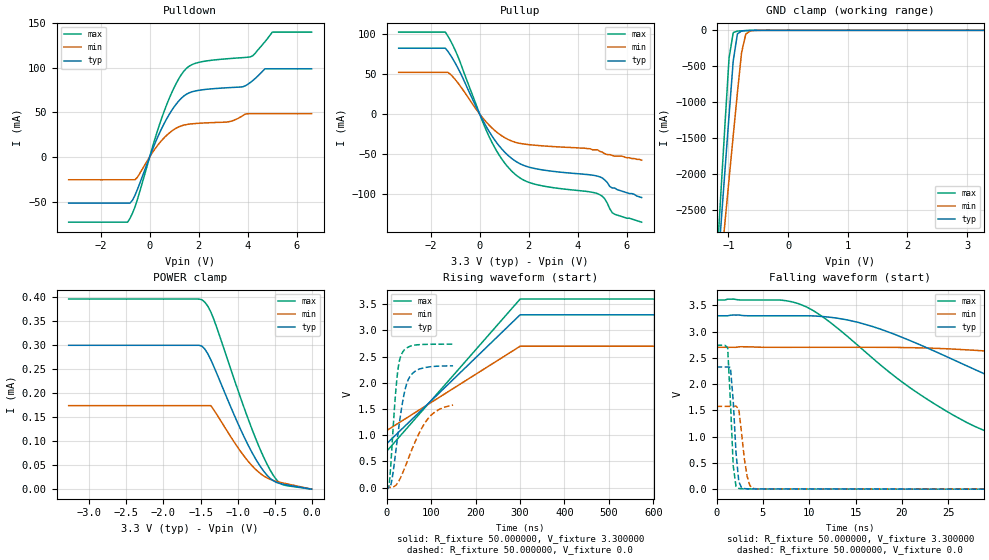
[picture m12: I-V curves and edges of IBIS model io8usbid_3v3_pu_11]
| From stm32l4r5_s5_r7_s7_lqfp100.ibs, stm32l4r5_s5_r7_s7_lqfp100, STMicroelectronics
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|   Model io8usbid_3v3_pu_11
[Model]  io8usbid_3v3_pu_11
Model_type I/O
Polarity   Non-Inverting
Enable   Active-Low
Vinl =   0.990000V
Vinh =   2.310000V
Vmeas =  1.650000V
Cref =   100.000000nF
Rref =   1.000000k
Vref =   3.300000V
C_comp   2.116400pF   2.092700pF   2.152900pF
[Temperature Range]   25.000000   0.125000k   -40.000000
[Pullup Reference]   3.300000V   2.700000V   3.600000V
[Pulldown Reference]   0.0V   0.0V   0.0V
[POWER Clamp Reference]   3.300000V   2.700000V   3.600000V
[GND Clamp Reference]   0.0V   0.0V   0.0V
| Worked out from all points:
|   slope of the pulldown table from 0 to 0.495 V, typ, clamps not added: 15.4 ohm
|   slope of the pullup table from 0 to 0.495 V, typ, clamps not added: 18.1 ohm
|   GND clamp passes 1 mA (typ) near -0.59 V on its own axis
|   rising waveform, R_fixture 50.000000, V_fixture 3.300000: 20-80 % time 180ns typ, 180ns min, 180ns max; typ from 0.836 V to 3.3 V
|   rising waveform, R_fixture 50.000000, V_fixture 0.0: 20-80 % time 23.9ns typ, 50.4ns min, 14.3ns max; typ from 0.001 V to 2.33 V
|   falling waveform, R_fixture 50.000000, V_fixture 3.300000: 20-80 % time 21ns typ, 41.6ns min, 13.6ns max; typ from 3.3 V to 0.836 V
|   falling waveform, R_fixture 50.000000, V_fixture 0.0: 20-80 % time 510ps typ, 662ps min, 429ps max; typ from 2.33 V to 0.001 V
[Pulldown]
|Voltage   I(typ)   I(min)   I(max)
-3.3V     -51.63mA   -25.53mA   -73.04mA
-900mV    -51.63mA   -25.53mA   -73.04mA
-500mV    -36.51mA   -22.79mA   -47.71mA
200mV     14.02mA    8.316mA    18.9mA
700mV     42.98mA    24.4mA     58.9mA
1.2V      63.06mA    33.8mA     88.14mA
1.6V      71.63mA    36.67mA    101.4mA
3.2V      77.51mA    39.29mA    110mA
4.1V      83.28mA    48.38mA    112mA
4.7V      98.63mA    48.38mA    129mA
5V        98.63mA    48.38mA    139.8mA
6.6V      98.63mA    48.43mA    139.8mA
[Pullup]
|Voltage   I(typ)   I(min)   I(max)
-3.3V     82.69mA    52.35mA    102.9mA
-1.4V     82.69mA    52.35mA    102.9mA
-900mV    58.56mA    39.63mA    73.37mA
100mV     -6.166mA   -3.962mA   -8.038mA
500mV     -27.53mA   -17.49mA   -35.6mA
1V        -47.29mA   -29.37mA   -60.81mA
1.5V      -60.05mA   -35.95mA   -77.15mA
2.4V      -69.45mA   -39.66mA   -89.34mA
4.8V      -78.1mA    -45mA      -100.1mA
5.1V      -83mA      -50mA      -106.7mA
5.5V      -93mA      -53mA      -126mA
6.6V      -105mA     -58mA      -136mA
[GND_clamp]
|Voltage   I(typ)   I(min)   I(max)
-3.3V     -9.914A    -9.595A    -9.188A
-1.2V     -3.541A    -3.911A    -3.279A
-1.13V    -2.75A     -3.295A    -2.301A
-1.06V    -1.963A    -2.68A     -1.33A
-990mV    -1.183A    -2.069A    -386.7mA
-920mV    -424.7mA   -1.463A    -31.42mA
-850mV    -49.12mA   -868.7mA   -10.48mA
-780mV    -9.121mA   -308.3mA   -6.715mA
-710mV    -3.648mA   -53.81mA   -3.986mA
-640mV    -1.726mA   -11.03mA   -1.885mA
-430mV    -22.46uA   -116.8uA   -9.748uA
3.28V     0A         0A         0A
[POWER_clamp]
|Voltage   I(typ)   I(min)   I(max)
-3.28V    299.3uA    173.7uA    395.4uA
-1.48V    297.5uA    173.7uA    393.9uA
-1.4V     281.3uA    173.7uA    380.3uA
-1.36V    268.9uA    173.7uA    368.3uA
-1.32V    255uA      164.8uA    353.1uA
-1.04V    152.4uA    96.77uA    226.2uA
-880mV    98.76uA    62.4uA     155.8uA
-720mV    53.77uA    36.12uA    92.05uA
-560mV    22.58uA    20.52uA    39.82uA
-480mV    14.4uA     16.42uA    20.64uA
-400mV    10.72uA    13.39uA    9.937uA
0V        0A         0A         0A
[Ramp]
| variable   typ   min   max
dV/dt_r  1.39450/23.89300n   0.94482/53.26837n   1.64288/14.28860n
dV/dt_f  1.47839/21.08553n   0.96684/44.67589n   1.74562/13.58476n
R_load = 50.000000
[Rising Waveform]
R_fixture= 50.000000
V_fixture= 3.300000
V_fixture_min= 2.700000
V_fixture_max= 3.600000
|time   V(typ)   V(min)   V(max)
0s        836mV      1.089V     690.6mV
300.3ns   3.3V       2.7V       3.6V
600.6ns   3.3V       2.7V       3.6V
29.73us   3.3V       2.7V       3.6V
[Rising Waveform]
R_fixture= 50.000000
V_fixture= 0.0
V_fixture_min= 0.0
V_fixture_max= 0.0
|time   V(typ)   V(min)   V(max)
0s        930.6uV    1.396mV    659.7uV
6.306ns   6.834mV    4.435mV    85.97mV
12.01ns   145.3mV    6.612mV    751.6mV
22.52ns   810mV      61.69mV    2.008V
28.23ns   1.193V     135.3mV    2.392V
33.03ns   1.476V     218.3mV    2.533V
43.54ns   1.934V     434.4mV    2.654V
58.56ns   2.183V     760.6mV    2.713V
97.3ns    2.307V     1.358V     2.737V
149.5ns   2.325V     1.576V     2.739V
[Falling Waveform]
R_fixture= 50.000000
V_fixture= 3.300000
V_fixture_min= 2.700000
V_fixture_max= 3.600000
|time   V(typ)   V(min)   V(max)
0s        3.3V       2.7V       3.6V
9.61ns    3.3V       2.7V       3.476V
15.32ns   3.173V     2.7V       2.726V
24.62ns   2.538V     2.673V     1.504V
29.13ns   2.177V     2.627V     1.101V
33.93ns   1.823V     2.554V     903.7mV
44.44ns   1.231V     2.33V      781mV
54.65ns   1.023V     2.075V     737.6mV
90.99ns   869.5mV    1.322V     697.4mV
149.5ns   836mV      1.089V     690.6mV
[Falling Waveform]
R_fixture= 50.000000
V_fixture= 0.0
V_fixture_min= 0.0
V_fixture_max= 0.0
|time   V(typ)   V(min)   V(max)
0s        2.325V     1.576V     2.739V
1.201ns   2.325V     1.576V     2.692V
1.502ns   2.318V     1.576V     1.659V
1.802ns   1.678V     1.576V     443.8mV
2.102ns   691.5mV    1.582V     54.51mV
2.402ns   146mV      1.527V     14.34mV
2.703ns   25.89mV    1.064V     8.518mV
3.604ns   6.757mV    66.36mV    5.733mV
4.505ns   5.615mV    6.846mV    5.077mV
149.5ns   930.6uV    1.396mV    659.7uV
